| Teraspeed Modeling Services.
| http://www.teraspeed.com
[IBIS Ver]   4.0
[Comment Char] |_char
[File Name]   lpc15xxjbd48.ibs
[File Rev]   3.0
[Source]  Measured and created by Teraspeed Consulting Group LLC
[Date]   03-05-2014
[Notes]   Quality Check of this IBIS model: Model Passes IBIS Check
   Model parses into ICX IS. Simulation done with Hyperlynx.
   1. MIN TYP MAX information is based on Temperature and Voltage
   characteristics only.
   2. Package data measured using Tektronix IConnect Software.
[Disclaimer]
| Use: Teraspeed Consulting Group LLC ("Teraspeed") has
| licensed IBIS models to specific integrated circuit
| suppliers ("IC Vendors") for use and distribution as
| follows: Each IC Vendor may use IBIS Models, and distribute
| them to IC Vendor's customers to use solely for developing
| printed circuit board designs. Users of this model may
| modify the IBIS model to suit its specific applications but
| rights to derivative works and such modifications shall belong
| to Teraspeed. No other distribution of these materials is
| permitted.
| DISCLAIMER OF WARRANTY: UNLESS OTHERWISE AGREED TO IN WRITING
| TERASPEED DISCLAIMS AND USER WAIVES ALL WARRANTIES, EXPRESS
| OR IMPLIED, INCLUDING WARRANTIES OF MERCHANTABILITY AND
| FITNESS FOR A PARTICULAR PURPOSE. IN NO EVENT SHALL
| TERASPEED BE LIABLE FOR ANY DIRECT OR INDIRECT DAMAGES,
| WHETHER IN CONTRACT OR TORT, INCLUDING, WITHOUT LIMITATION,
| LOST PROFITS, BUSINESS INTERRUPTION, OR LOST INFORMATION
| ARISING OUT OF THE USE OF OR THE INABILITY TO USE THE MODEL,
| EVEN IF TERASPEED HAS BEEN ADVISED OF THE POSSIBILITY OF SUCH
| DAMAGES.
[Copyright]
| This file is the legal property of Teraspeed Copyright(c) 2014.
| All other rights are reserved.
[Component]LPC15xxJBD48
[Manufacturer] NXP Semiconductors
[Package]
| variable   typ   min   max
| qfp48
R_pkg  1.68E-02 1.487E-02   1.887E-02
L_pkg  2.02E-09 1.784E-09   2.264E-09
C_pkg  5.61E-13 4.955E-13   6.289E-13
[Pin] signal_name  model_name  R_pin  L_pin C_pin
1   PIO0_0   pio0_0   0.0189  2.264E-09   6.289E-13
2   PIO0_1   pio0_1   0.0180  2.163E-09   6.009E-13
3   PIO0_2   pio0_2   0.0172  2.065E-09   5.735E-13
4   PIO0_3   pio0_3   0.0164  1.968E-09   5.467E-13
5   PIO0_4   pio0_4   0.0156  1.874E-09   5.207E-13
6   PIO0_5   pio0_5   0.0149  1.784E-09   4.955E-13
7   PIO0_6   pio0_6   0.0149  1.784E-09   4.955E-13
8   PIO0_7   pio0_7   0.0156  1.874E-09   5.207E-13
9   PIO0_8   pio0_8   0.0164  1.968E-09   5.467E-13
10   VREFP_ADC   POWER   0.0172  2.065E-09   5.735E-13
11   VREFN   POWER   0.0180  2.163E-09   6.009E-13
12   PIO0_9   pio0_9   0.0189  2.264E-09   6.289E-13
13   PIO0_18   pio0_18   0.0189  2.264E-09   6.289E-13
14   VREFP_DAC_VDDCMP POWER  0.0180  2.163E-09   6.009E-13
15   PIO0_10   pio0_10   0.0172  2.065E-09   5.735E-13
16   VDDA   POWER   0.0164  1.968E-09   5.467E-13
17   VSSA   GND   0.0156  1.874E-09   5.207E-13
18   PIO0_11   pio0_11   0.0149  1.784E-09   4.955E-13
19   PIO0_12   pio0_12   0.0149  1.784E-09   4.955E-13
20   VSS   GND   0.0156  1.874E-09   5.207E-13
21   PIO0_13   pio0_13   0.0164  1.968E-09   5.467E-13
22   PIO0_14   pio0_14   0.0172  2.065E-09   5.735E-13
23   PIO0_15   pio0_15   0.0180  2.163E-09   6.009E-13
24   PIO0_16   pio0_16   0.0189  2.264E-09   6.289E-13
25   XTALOUT   term   0.0189  2.264E-09   6.289E-13
26   XTALIN   xtalin   0.0180  2.163E-09   6.009E-13
27   VDD   POWER   0.0172  2.065E-09   5.735E-13
28   PIO0_17   pio0_17   0.0164  1.968E-09   5.467E-13
29   PIO0_19   pio0_19   0.0156  1.874E-09   5.207E-13
30   VBAT   POWER   0.0149  1.784E-09   4.955E-13
31   RTCXIN   rtcxin   0.0149  1.784E-09   4.955E-13
32   RTCXOUT   rtcxout   0.0156  1.874E-09   5.207E-13
33   PIO0_20   pio0_20   0.0164  1.968E-09   5.467E-13
34   RESET   pio0_21   0.0172  2.065E-09   5.735E-13
35   USB_DP   usb   0.0180  2.163E-09   6.009E-13
36   USB_DM   usb   0.0189  2.264E-09   6.289E-13
37   PIO0_22   pio0_22   0.0189  2.264E-09   6.289E-13
38   PIO0_23   pio0_23   0.0180  2.163E-09   6.009E-13
39   VDD   POWER   0.0172  2.065E-09   5.735E-13
40   VSS   GND   0.0164  1.968E-09   5.467E-13
41   VSS   GND   0.0156  1.874E-09   5.207E-13
42   VDD   POWER   0.0149  1.784E-09   4.955E-13
43   PIO0_24   pio0_24   0.0149  1.784E-09   4.955E-13
44   PIO0_25   pio0_25   0.0156  1.874E-09   5.207E-13
45   PIO0_26   pio0_26   0.0164  1.968E-09   5.467E-13
46   PIO0_27   pio0_27   0.0172  2.065E-09   5.735E-13
47   PIO0_28   pio0_28   0.0180  2.163E-09   6.009E-13
48   PIO0_29   pio0_29   0.0189  2.264E-09   6.289E-13
[Model Selector]   pio0_0
pio_2.5v   GP io 2.5V
pio_3.3v   GP io 3.3V
pio_2.5v_pu   GP io 2.5V with pullup
pio_3.3v_pu   GP io 3.3V with pullup
pio_2.5v_pd   GP io 2.5V with pulldown
pio_3.3v_pd   GP io 3.3V with pulldown
[Model Selector]   pio0_1
pio_2.5v   GP io 2.5V
pio_3.3v   GP io 3.3V
pio_2.5v_pu   GP io 2.5V with pullup
pio_3.3v_pu   GP io 3.3V with pullup
pio_2.5v_pd   GP io 2.5V with pulldown
pio_3.3v_pd   GP io 3.3V with pulldown
[Model Selector]   pio0_2
pio_2.5v   GP io 2.5V
pio_3.3v   GP io 3.3V
pio_2.5v_pu   GP io 2.5V with pullup
pio_3.3v_pu   GP io 3.3V with pullup
pio_2.5v_pd   GP io 2.5V with pulldown
pio_3.3v_pd   GP io 3.3V with pulldown
[Model Selector]   pio0_3
pio_2.5v   GP io 2.5V
pio_3.3v   GP io 3.3V
pio_2.5v_pu   GP io 2.5V with pullup
pio_3.3v_pu   GP io 3.3V with pullup
pio_2.5v_pd   GP io 2.5V with pulldown
pio_3.3v_pd   GP io 3.3V with pulldown
[Model Selector]   pio0_4
pio_2.5v   GP io 2.5V
pio_3.3v   GP io 3.3V
pio_2.5v_pu   GP io 2.5V with pullup
pio_3.3v_pu   GP io 3.3V with pullup
pio_2.5v_pd   GP io 2.5V with pulldown
pio_3.3v_pd   GP io 3.3V with pulldown
[Model Selector]   pio0_5
pio_2.5v   GP io 2.5V
pio_3.3v   GP io 3.3V
pio_2.5v_pu   GP io 2.5V with pullup
pio_3.3v_pu   GP io 3.3V with pullup
pio_2.5v_pd   GP io 2.5V with pulldown
pio_3.3v_pd   GP io 3.3V with pulldown
[Model Selector]   pio0_6
pio_2.5v   GP io 2.5V
pio_3.3v   GP io 3.3V
pio_2.5v_pu   GP io 2.5V with pullup
pio_3.3v_pu   GP io 3.3V with pullup
pio_2.5v_pd   GP io 2.5V with pulldown
pio_3.3v_pd   GP io 3.3V with pulldown
[Model Selector]   pio0_7
pio_2.5v   GP io 2.5V
pio_3.3v   GP io 3.3V
pio_2.5v_pu   GP io 2.5V with pullup
pio_3.3v_pu   GP io 3.3V with pullup
pio_2.5v_pd   GP io 2.5V with pulldown
pio_3.3v_pd   GP io 3.3V with pulldown
[Model Selector]   pio0_8
pio_2.5v   GP io 2.5V
pio_3.3v   GP io 3.3V
pio_2.5v_pu   GP io 2.5V with pullup
pio_3.3v_pu   GP io 3.3V with pullup
pio_2.5v_pd   GP io 2.5V with pulldown
pio_3.3v_pd   GP io 3.3V with pulldown
[Model Selector]   pio0_9
pio_2.5v   GP io 2.5V
pio_3.3v   GP io 3.3V
pio_2.5v_pu   GP io 2.5V with pullup
pio_3.3v_pu   GP io 3.3V with pullup
pio_2.5v_pd   GP io 2.5V with pulldown
pio_3.3v_pd   GP io 3.3V with pulldown
[Model Selector]   pio0_10
pio_2.5v   GP io 2.5V
pio_3.3v   GP io 3.3V
pio_2.5v_pu   GP io 2.5V with pullup
pio_3.3v_pu   GP io 3.3V with pullup
pio_2.5v_pd   GP io 2.5V with pulldown
pio_3.3v_pd   GP io 3.3V with pulldown
[Model Selector]   pio0_11
pio_2.5v   GP io 2.5V
pio_3.3v   GP io 3.3V
pio_2.5v_pu   GP io 2.5V with pullup
pio_3.3v_pu   GP io 3.3V with pullup
pio_2.5v_pd   GP io 2.5V with pulldown
pio_3.3v_pd   GP io 3.3V with pulldown
[Model Selector]   pio0_12
pio_2.5v   GP io 2.5V
pio_3.3v   GP io 3.3V
pio_2.5v_pu   GP io 2.5V with pullup
pio_3.3v_pu   GP io 3.3V with pullup
pio_2.5v_pd   GP io 2.5V with pulldown
pio_3.3v_pd   GP io 3.3V with pulldown
[Model Selector]   pio0_13
pio_2.5v   GP io 2.5V
pio_3.3v   GP io 3.3V
pio_2.5v_pu   GP io 2.5V with pullup
pio_3.3v_pu   GP io 3.3V with pullup
pio_2.5v_pd   GP io 2.5V with pulldown
pio_3.3v_pd   GP io 3.3V with pulldown
[Model Selector]   pio0_14
pio_2.5v   GP io 2.5V
pio_3.3v   GP io 3.3V
pio_2.5v_pu   GP io 2.5V with pullup
pio_3.3v_pu   GP io 3.3V with pullup
pio_2.5v_pd   GP io 2.5V with pulldown
pio_3.3v_pd   GP io 3.3V with pulldown
[Model Selector]   pio0_15
pio_2.5v   GP io 2.5V
pio_3.3v   GP io 3.3V
pio_2.5v_pu   GP io 2.5V with pullup
pio_3.3v_pu   GP io 3.3V with pullup
pio_2.5v_pd   GP io 2.5V with pulldown
pio_3.3v_pd   GP io 3.3V with pulldown
[Model Selector]   pio0_16
pio_2.5v   GP io 2.5V
pio_3.3v   GP io 3.3V
pio_2.5v_pu   GP io 2.5V with pullup
pio_3.3v_pu   GP io 3.3V with pullup
pio_2.5v_pd   GP io 2.5V with pulldown
pio_3.3v_pd   GP io 3.3V with pulldown
[Model Selector]   pio0_17
pio_2.5v   GP io 2.5V
pio_3.3v   GP io 3.3V
pio_2.5v_pu   GP io 2.5V with pullup
pio_3.3v_pu   GP io 3.3V with pullup
pio_2.5v_pd   GP io 2.5V with pulldown
pio_3.3v_pd   GP io 3.3V with pulldown
[Model Selector]   pio0_18
pio_2.5v   GP io 2.5V
pio_3.3v   GP io 3.3V
pio_2.5v_pu   GP io 2.5V with pullup
pio_3.3v_pu   GP io 3.3V with pullup
pio_2.5v_pd   GP io 2.5V with pulldown
pio_3.3v_pd   GP io 3.3V with pulldown
[Model Selector]   pio0_19
pio_2.5v   GP io 2.5V
pio_3.3v   GP io 3.3V
pio_2.5v_pu   GP io 2.5V with pullup
pio_3.3v_pu   GP io 3.3V with pullup
pio_2.5v_pd   GP io 2.5V with pulldown
pio_3.3v_pd   GP io 3.3V with pulldown
[Model Selector]   pio0_20
pio_2.5v   GP io 2.5V
pio_3.3v   GP io 3.3V
pio_2.5v_pu   GP io 2.5V with pullup
pio_3.3v_pu   GP io 3.3V with pullup
pio_2.5v_pd   GP io 2.5V with pulldown
pio_3.3v_pd   GP io 3.3V with pulldown
[Model Selector]   pio0_21
pio_2.5v   GP io 2.5V
pio_3.3v   GP io 3.3V
pio_2.5v_pu   GP io 2.5V with pullup
pio_3.3v_pu   GP io 3.3V with pullup
pio_2.5v_pd   GP io 2.5V with pulldown
pio_3.3v_pd   GP io 3.3V with pulldown
resetb_in_2.5v  2.5V reset input
resetb_in_3.3v  3.3V reset input
[Model Selector]   pio0_22
pio_2.5v   GP io 2.5V
pio_3.3v   GP io 3.3V
pio_2.5v_pu   GP io 2.5V with pullup
pio_3.3v_pu   GP io 3.3V with pullup
pio_2.5v_pd   GP io 2.5V with pulldown
pio_3.3v_pd   GP io 3.3V with pulldown
i2c_std_fst_2.5v   I2C Open Drain io 2.5V
i2c_std_fst_3.3v   I2C Open Drain io 3.3V
[Model Selector]   pio0_23
pio_2.5v   GP io 2.5V
pio_3.3v   GP io 3.3V
pio_2.5v_pu   GP io 2.5V with pullup
pio_3.3v_pu   GP io 3.3V with pullup
pio_2.5v_pd   GP io 2.5V with pulldown
pio_3.3v_pd   GP io 3.3V with pulldown
i2c_std_fst_2.5v   I2C Open Drain io 2.5V
i2c_std_fst_3.3v   I2C Open Drain io 3.3V
[Model Selector]   pio0_24
hd_pio_2.5v   High Drive GP io 2.5V
hd_pio_3.3v   High Drive GP io 3.3V
hd_pio_2.5v_pu   High Drive GP io 2.5V with pullup
hd_pio_3.3v_pu   High Drive GP io 3.3V with pullup
hd_pio_2.5v_pd   High Drive GP io 2.5V with pulldown
hd_pio_3.3v_pd   High Drive GP io 3.3V with pulldown
[Model Selector]   pio0_25
pio_2.5v   GP io 2.5V
pio_3.3v   GP io 3.3V
pio_2.5v_pu   GP io 2.5V with pullup
pio_3.3v_pu   GP io 3.3V with pullup
pio_2.5v_pd   GP io 2.5V with pulldown
pio_3.3v_pd   GP io 3.3V with pulldown
[Model Selector]   pio0_26
pio_2.5v   GP io 2.5V
pio_3.3v   GP io 3.3V
pio_2.5v_pu   GP io 2.5V with pullup
pio_3.3v_pu   GP io 3.3V with pullup
pio_2.5v_pd   GP io 2.5V with pulldown
pio_3.3v_pd   GP io 3.3V with pulldown
[Model Selector]   pio0_27
pio_2.5v   GP io 2.5V
pio_3.3v   GP io 3.3V
pio_2.5v_pu   GP io 2.5V with pullup
pio_3.3v_pu   GP io 3.3V with pullup
pio_2.5v_pd   GP io 2.5V with pulldown
pio_3.3v_pd   GP io 3.3V with pulldown
[Model Selector]   pio0_28
pio_2.5v   GP io 2.5V
pio_3.3v   GP io 3.3V
pio_2.5v_pu   GP io 2.5V with pullup
pio_3.3v_pu   GP io 3.3V with pullup
pio_2.5v_pd   GP io 2.5V with pulldown
pio_3.3v_pd   GP io 3.3V with pulldown
[Model Selector]   pio0_29
pio_2.5v   GP io 2.5V
pio_3.3v   GP io 3.3V
pio_2.5v_pu   GP io 2.5V with pullup
pio_3.3v_pu   GP io 3.3V with pullup
pio_2.5v_pd   GP io 2.5V with pulldown
pio_3.3v_pd   GP io 3.3V with pulldown
[Model Selector]   rtcxin
rtcx_2.5v   Real Time Clock 2.5V input
rtcx_3.3v   Real Time Clock 3.3V input
[Model Selector]   rtcxout
out_2.5v   Real Time Clock 2.5V output
out_3.3v   Real Time Clock 3.3V output
[Model Selector]   usb
usb1_np_2.5v   usb1 io,np,2.5v
usb1_np_3.3v   usb1 io,np,3.3v
usb1_pd_2.5v   usb1 io,pd,2.5v
usb1_pd_3.3v   usb1 io,pd,3.3v
[Model Selector] xtalin
xtal_2.5v   2.5V crystal osc input
xtal_3.3v   3.3V crystal osc input
[Model] term
Model_type Terminator
C_comp  0pF 0pF 0pF
| variable typ   min   max
[Voltage Range]   3.30000V  3.00000V  3.60000V
[POWER Clamp Reference]  3.30000V  3.00000V  3.60000V
[GND Clamp Reference]   0.00000V  0.00000V  0.00000V
[Temperature Range]   25   85   -40
| Models and submodels in the file (27): hd_pio_2.5v (Input), hd_pio_2.5v_pd (Input), hd_pio_2.5v_pu (Input), hd_pio_3.3v (Input), hd_pio_3.3v_pd (Input), hd_pio_3.3v_pu (Input), pio_2.5v (Input), pio_2.5v_pd (Input), pio_2.5v_pu (Input), pio_3.3v (Input), pio_3.3v_pd (Input), pio_3.3v_pu (Input), resetb_in_2.5v (Input), resetb_in_3.3v (Input), rtcx_2.5v (Input), rtcx_3.3v (Input), xtal_2.5v (Input), xtal_3.3v (Input), i2c_std_fst_2.5v (I/O_open_drain), i2c_std_fst_3.3v (I/O_open_drain), usb1_np_2.5v (I/O), usb1_pd_2.5v (I/O), usb1_np_3.3v (I/O), usb1_pd_3.3v (I/O), out_2.5v (I/O), out_3.3v (I/O), term (Terminator)
